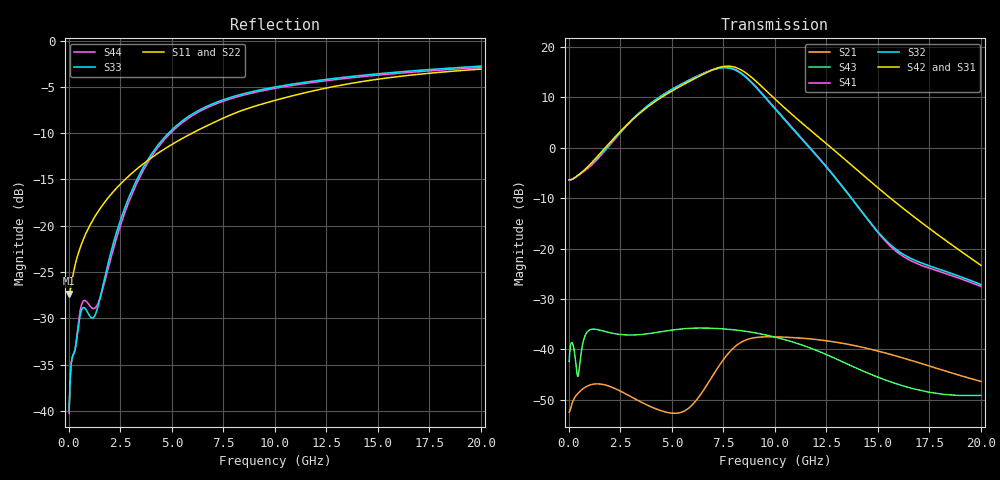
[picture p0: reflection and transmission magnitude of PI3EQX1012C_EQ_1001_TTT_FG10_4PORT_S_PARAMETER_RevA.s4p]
! NPort=4 DATA=2000 NOISE=0 GROUPDELAY=0 COMPLEX_DATAFORMAT=POLAR
! NumOfBlock=1 NumOfParam=0
! .MODEL Smodel S TSTONEFILE=PI3EQX1012C_EQ_1001_TTT_FG10_4PORT_S_PARAMETER_RevA.s4p TYPE=S
!  -- The above .MODEL line can be used for the S element in the netlist.
! The s parameter is extracted from the linear redriver, it is not bi-directional; only s(4,1)s(4,2) and s(3,1)s(3,2)
! should be the insertion loss
!Port definition:
!Port1 = input+
!Port2 = input-
!Port3 = output+
!Port4 = output-
# Hz S MA R  50
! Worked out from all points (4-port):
!   2000 points, 10 MHz to 20 GHz, reference 50 ohm
!   strongest paths, dB at 10 MHz, 5.01 GHz, 10.01 GHz, 15.01 GHz, 20 GHz:
!     S42: -6.4, 11.2, 9.6, -8.0, -23.3
!     S31: -6.4, 11.2, 9.5, -8.2, -23.8
!     S32: -6.4, 11.6, 7.6, -16.7, -27.1
!     S41: -6.4, 11.6, 7.8, -16.9, -27.5
!     S43: -42.4, -36.2, -37.6, -45.5, -49.1
!     S21: -52.4, -52.6, -37.5, -40.3, -46.3
!   lowest |S11| = -27.3 dB at 10 MHz (marker M1), VSWR 1.09, Z = 45.9 - j0.123 ohm
!   |S11| at or under -10 dB: start of sweep to 5.985 GHz
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1e7  0.04301 -178.2  0.002379 1.5  0.0008102 -0.5  0.0008039 -0.5
     0.002388 1.5  0.04109 -178.1  0.000927 -0.5  0.0009197 -0.5
     0.4785 0.0  0.4777 -179.9  0.01016 -4.0  0.007598 -25.7
     0.4772 -179.9  0.4795 -0.0  0.007614 -25.8  0.009722 -4.0
4.14e9  0.2385 -124.3  0.002637 1.3  0.000378 -57.0  0.0003763 -57.4
        0.002618 1.3  0.2422 -123.1  0.0004297 -57.7  0.0004277 -58.0
        2.819 -62.9  2.911 126.6  0.2561 -84.0  0.01369 33.3
        2.897 127.3  2.817 -61.2  0.01461 30.1  0.2483 -83.7
5.83e9  0.3097 -123.7  0.002731 48.7  0.0002743 -58.2  0.0002731 -59.2
        0.002633 46.6  0.3148 -123.1  0.0003109 -59.2  0.0003097 -60.1
        4.49 -131.5  4.643 57.5  0.3906 -100.1  0.01649 8.2
        4.661 57.7  4.51 -129.6  0.01617 5.6  0.3828 -99.9
7.11e9  0.3644 -124.3  0.006363 65.6  0.0002384 -55.8  0.0002363 -57.1
        0.006045 66.5  0.3698 -123.8  0.0002689 -57.0  0.0002666 -58.3
        6.009 165.2  5.989 -6.7  0.4618 -109.9  0.01671 -11.7
        6.039 -6.8  6.045 167.3  0.01616 -12.5  0.4536 -109.8
8.15e9  0.4092 -125.8  0.01136 44.7  0.0002242 -54.2  0.0002211 -55.7
        0.01102 46.3  0.4151 -125.3  0.0002512 -55.5  0.0002479 -57.0
        6.127 100.7  5.767 -71.7  0.5046 -116.1  0.01587 -26.0
        5.833 -72.1  6.167 103.0  0.01553 -26.1  0.4959 -116.0
9.32e9  0.4523 -127.9  0.01348 14.9  0.0002153 -53.8  0.0002113 -55.4
        0.01327 16.4  0.4592 -127.5  0.0002397 -55.0  0.0002355 -56.6
        4.076 34.2  3.498 -137.8  0.5423 -121.6  0.01449 -40.0
        3.549 -138.7  4.104 36.8  0.01424 -40.5  0.5336 -121.4
2e10  0.7008 -144.6  0.004876 -73.9  0.0001464 -72.3  0.0001413 -73.8
      0.004826 -72.8  0.7158 -144.4  0.0001624 -72.1  0.0001566 -73.8
      0.06484 103.4  0.04391 30.6  0.7272 -143.5  0.003588 -51.5
      0.04212 28.9  0.06815 108.2  0.003506 -48.9  0.7152 -143.3
